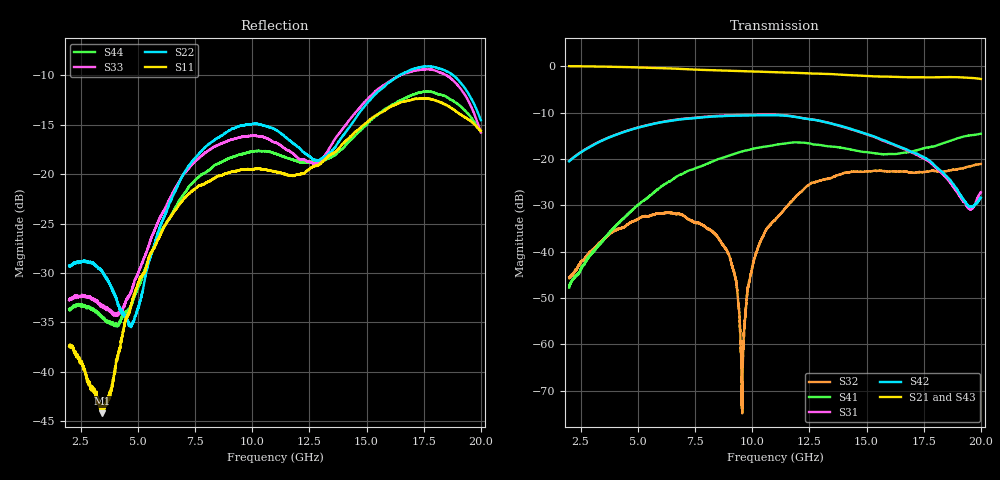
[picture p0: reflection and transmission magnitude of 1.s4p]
!Keysight Technologies,N5225A,MY51451420,A.10.40.12
!Date: Thursday, October 15, 2015 10:00:10
!Correction: S11(Full 4 Port(1,2,3,4))
!S12(Full 4 Port(1,2,3,4))
!S13(Full 4 Port(1,2,3,4))
!S14(Full 4 Port(1,2,3,4))
!S21(Full 4 Port(1,2,3,4))
!S22(Full 4 Port(1,2,3,4))
!S23(Full 4 Port(1,2,3,4))
!S24(Full 4 Port(1,2,3,4))
!S31(Full 4 Port(1,2,3,4))
!S32(Full 4 Port(1,2,3,4))
!S33(Full 4 Port(1,2,3,4))
!S34(Full 4 Port(1,2,3,4))
!S41(Full 4 Port(1,2,3,4))
!S42(Full 4 Port(1,2,3,4))
!S43(Full 4 Port(1,2,3,4))
!S44(Full 4 Port(1,2,3,4))
!S4P File: Measurements: <S11,S12,S13,S14>,
!<S21,S22,S23,S24>,
!<S31,S32,S33,S34>,
!<S41,S42,S43,S44>:
# Hz S  dB  R 50
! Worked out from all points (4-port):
!   6401 points, 2 GHz to 20 GHz, reference 50 ohm
!   strongest paths, dB at 2 GHz, 6.5 GHz, 11 GHz, 15.5 GHz, 20 GHz:
!     S21: 0.1, -0.4, -1.2, -2.2, -2.7
!     S43: 0.0, -0.5, -1.3, -2.3, -2.6
!     S42: -20.5, -11.7, -10.5, -15.4, -28.3
!     S31: -20.4, -11.6, -10.4, -15.6, -27.1
!     S41: -47.8, -24.5, -17.0, -18.8, -14.5
!     S32: -45.6, -31.7, -33.2, -22.5, -21.1
!   lowest |S11| = -44.2 dB at 3.454 GHz (marker M1), VSWR 1.01, Z = 50.5 - j0.303 ohm
!   |S11| at or under -10 dB: start of sweep to end of sweep
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2e9  -37.40 78.1  0.06 -39.1  -20.41 50.7  -47.60 62.1
     0.06 -39.1  -29.26 70.0  -45.54 110.2  -20.47 50.7
     -20.42 50.6  -45.59 110.7  -32.74 70.4  -0.03 -39.3
     -47.75 62.4  -20.48 50.7  -0.03 -39.2  -33.68 36.6
3.454062e9  -44.21 -29.1  -0.03 -67.5  -15.93 22.3  -37.85 7.3
            -0.04 -67.6  -29.84 49.2  -37.56 70.4  -15.99 22.5
            -15.93 22.3  -37.58 70.5  -33.28 69.3  -0.12 -67.7
            -37.81 7.6  -15.98 22.5  -0.12 -67.8  -34.49 -27.3
8.26625e9  -20.53 94.0  -0.81 -161.1  -10.74 -73.5  -20.53 -160.2
           -0.81 -161.1  -16.71 99.0  -35.72 -81.9  -10.84 -73.4
           -10.74 -73.5  -35.66 -81.8  -17.33 95.0  -0.85 -161.7
           -20.52 -160.3  -10.83 -73.4  -0.85 -161.7  -19.31 95.9
9.562812e9  -19.56 53.2  -1.02 174.0  -10.48 -99.0  -18.37 158.2
            -1.02 173.9  -15.06 80.4  -71.58 -2.5  -10.62 -98.6
            -10.48 -99.1  -71.99 -28.3  -16.22 77.9  -1.04 173.3
            -18.37 158.1  -10.62 -98.6  -1.04 173.3  -17.96 58.7
1.025188e10  -19.46 28.6  -1.13 160.6  -10.43 -112.8  -17.56 136.1
             -1.13 160.6  -14.92 70.8  -39.14 25.1  -10.56 -112.0
             -10.43 -112.8  -39.21 24.5  -16.14 69.9  -1.15 159.8
             -17.56 136.1  -10.56 -112.0  -1.15 159.8  -17.66 36.3
1.238094e10  -19.69 -72.2  -1.47 119.0  -11.29 -158.3  -16.54 69.5
             -1.47 118.9  -18.01 62.3  -25.88 -36.8  -11.32 -157.2
             -11.29 -158.3  -25.91 -36.6  -18.70 70.1  -1.53 117.6
             -16.55 69.4  -11.31 -157.2  -1.53 117.6  -18.79 -54.8
2e10  -15.63 -33.1  -2.71 -42.3  -27.13 155.9  -14.51 -80.5
      -2.71 -42.4  -14.53 16.9  -21.06 142.7  -28.29 150.0
      -27.13 155.9  -21.06 142.7  -15.78 7.0  -2.62 -43.2
      -14.53 -80.6  -28.32 150.3  -2.63 -43.2  -15.73 -15.5
